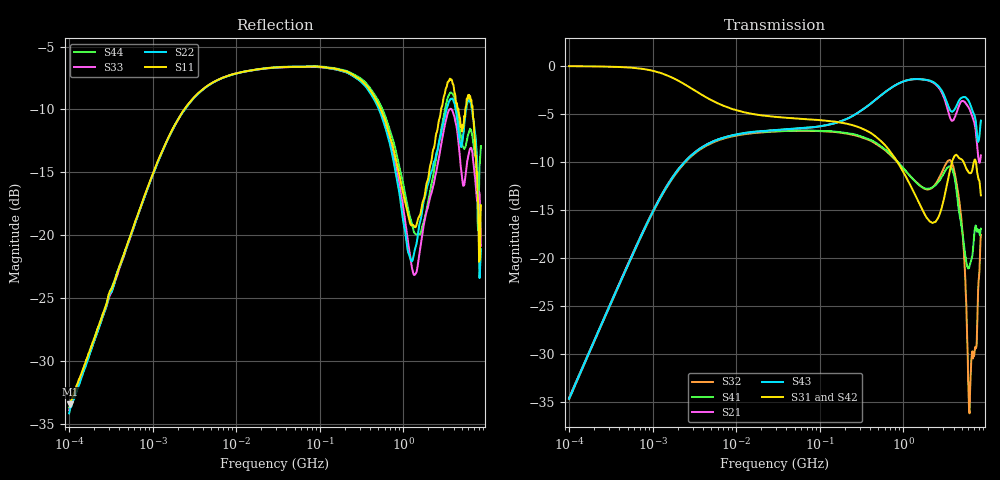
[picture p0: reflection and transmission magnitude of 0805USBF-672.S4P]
# Hz S dB R 50
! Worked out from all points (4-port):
!   801 points, 100 kHz to 8.5 GHz, reference 50 ohm
!   strongest paths, dB at 100 kHz, 1.721 MHz, 29.51 MHz, 502.3 MHz, 8.5 GHz:
!     S31: -0.1, -1.3, -5.3, -7.6, -13.5
!     S42: 0.0, -1.2, -5.3, -7.6, -13.8
!     S43: -34.7, -11.7, -6.7, -3.3, -5.7
!     S21: -34.6, -11.6, -6.7, -3.3, -9.3
!     S41: -34.6, -11.7, -6.8, -8.2, -17.0
!     S32: -34.7, -11.8, -6.9, -8.3, -17.6
!   lowest |S11| = -33.5 dB at 101.7 kHz (marker M1), VSWR 1.04, Z = 50.5 + j2.09 ohm
!   |S11| at or under -10 dB: 537.5 MHz to 2.838 GHz (2.301 GHz wide, 136 % of centre); 4.575 GHz to 5.533 GHz (958 MHz wide, 19 % of centre); 6.769 GHz to end of sweep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
100000  -33.46 76.3  -34.62 86.9  -0.07 -1.1  -34.70 -92.9
        -34.59 86.9  -34.19 75.1  -34.78 -92.8  -0.04 -1.0
        -0.07 -1.1  -34.73 -92.9  -33.93 69.9  -34.67 87.1
        -34.62 -93.2  -0.04 -1.0  -34.68 87.1  -33.73 77.1
101665  -33.46 76.6  -34.46 87.0  -0.07 -1.1  -34.55 -93.0
        -34.45 86.9  -33.96 75.0  -34.63 -92.9  -0.04 -1.1
        -0.07 -1.1  -34.56 -93.0  -33.80 69.8  -34.53 87.1
        -34.48 -93.2  -0.04 -1.0  -34.53 86.9  -33.63 77.8
7.175618e8  -12.45 -138.6  -2.31 -100.6  -9.09 -172.6  -9.30 4.3
            -2.32 -100.6  -13.20 -144.9  -9.41 -0.8  -9.03 -172.7
            -9.09 -172.6  -9.41 -0.8  -12.80 -146.5  -2.32 -99.3
            -9.29 4.3  -9.02 -172.6  -2.32 -99.3  -11.97 -140.8
1.686463e9  -17.55 127.6  -1.43 89.0  -14.97 -8.9  -12.67 171.7
            -1.44 89.0  -18.08 144.6  -12.66 164.5  -15.10 -8.6
            -14.97 -8.9  -12.66 164.5  -20.03 138.2  -1.44 92.4
            -12.67 171.6  -15.12 -8.7  -1.44 92.3  -19.34 118.0
2.726397e9  -10.69 -45.2  -2.43 -89.7  -15.47 141.4  -11.97 -22.2
            -2.43 -89.8  -12.43 -24.1  -11.61 -23.4  -15.56 145.5
            -15.50 141.4  -11.61 -23.4  -13.48 -32.2  -2.29 -83.7
            -11.95 -22.3  -15.54 145.5  -2.30 -83.7  -12.30 -43.2
3.88629e9  -7.91 93.0  -5.73 92.3  -9.89 -117.6  -10.89 88.9
           -5.75 92.2  -9.15 98.2  -10.28 93.6  -10.32 -115.0
           -9.88 -117.7  -10.28 93.7  -10.11 103.8  -4.79 98.4
           -10.86 88.8  -10.31 -115.0  -4.80 98.4  -8.74 102.1
8.5e9  -17.63 65.6  -9.33 78.7  -13.56 74.8  -16.92 164.5
       -9.35 78.3  -21.13 90.9  -17.75 -178.5  -13.77 73.1
       -13.51 74.8  -17.62 -178.5  -20.86 64.8  -5.74 85.2
       -16.98 165.4  -13.78 72.8  -5.73 85.2  -12.93 60.0
